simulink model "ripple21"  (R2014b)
settings: Solver=ode45  StartTime=0.0  StopTime=10.0  RelTol=1e-3
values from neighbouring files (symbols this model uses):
  h = firls(n, f, a, wi)    [fir_ls_1.m]    (also in fir_pm_2.m = firpm(n, f0, a0, wi); fir_pm_3.m = firpm(n, f0, a0, wi); ideale_filter_4.m = fir1(N, [fs1, fs2]*2/fs, 'stop', hamming(N+1)); inv_sinc_1.m = hd)
  hTP = fir1(128, 0.2)    [ripple_21.m]
  nbit = 16    [ripple_21.m]
  nord = 18    [fdesign_1.m]    (also in grp_komp_1.m = 6; hilbert_filter_1.m = 64; hilbert_filter_2.m = 64; hilbert_filter_3.m = 64)
  Ts = 1/fs    (= 0.001)    [abtast_fir_1.m]    (also in abtast_fir_2.m; abtast_fir_3.m; abtast_fir_4.m; hilbert_filter_1.m)
libraries: dspstat3 x2, simulink x1

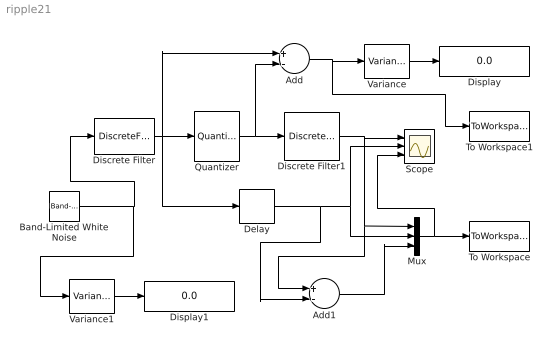
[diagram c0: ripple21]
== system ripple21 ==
  Add : Sum  Inputs=+-
  Add1 : Sum  Inputs=+-
  Band-Limited White Noise : simulink/Sources/Band-Limited White Noise  Cov=Ts  Ts=Ts  seed=[23341]
  Delay : Delay  DelayLength=nord/2
  Discrete Filter : DiscreteFilter  Numerator=hTP  Denominator=1
  Discrete Filter1 : DiscreteFilter  Numerator=h  Denominator=1
  Display : Display
  Display1 : Display
  Mux : Mux  Inputs=3
  Quantizer : Quantizer  QuantizationInterval=1/(2^nbit)
  Scope : Scope  NumInputPorts=3
  To Workspace : ToWorkspace  VariableName=y  SaveFormat=Timeseries  SampleTime=-1
  To Workspace1 : ToWorkspace  VariableName=y1  SaveFormat=Timeseries  SampleTime=-1
  Variance : dspstat3/Variance  run=on  reset_popup=None  InputProcessing=Columns as channels (frame based)  directionMode=Each column  dimension=1  treatSBRowAsCol=on  roiEnable=off  roiType=Rectangles  roiPortion=Entire ROI  roiOutput=Individual statistics for each ROI  roiFlag=off  roundingMode=Floor  overflowMode=off
  Variance1 : dspstat3/Variance  run=on  reset_popup=None  InputProcessing=Columns as channels (frame based)  directionMode=Each column  dimension=1  treatSBRowAsCol=on  roiEnable=off  roiType=Rectangles  roiPortion=Entire ROI  roiOutput=Individual statistics for each ROI  roiFlag=off  roundingMode=Floor  overflowMode=off
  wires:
  Quantizer/1 -> Add/2, Discrete Filter1/1
  Add/1 -> To Workspace1/1, Variance/1
  Variance/1 -> Display/1
  Delay/1 -> Add1/2, Mux/2, Scope/2
  Mux/1 -> To Workspace/1, Scope/3
  Add1/1 -> Mux/3
  Discrete Filter1/1 -> Mux/1, Add1/1, Scope/1
  Discrete Filter/1 -> Delay/1, Add/1, Quantizer/1
  Band-Limited White Noise/1 -> Variance1/1, Discrete Filter/1
  Variance1/1 -> Display1/1
